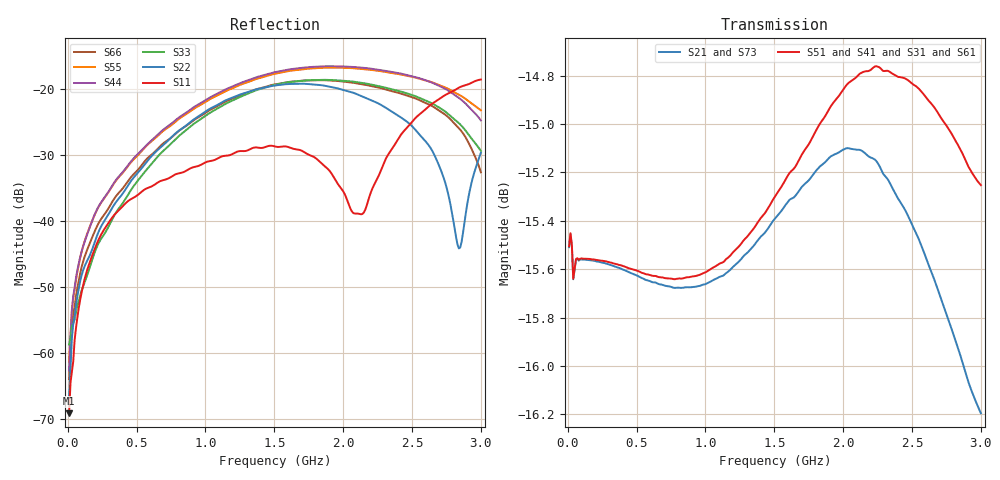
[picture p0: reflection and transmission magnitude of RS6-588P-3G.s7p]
! MTS Systemtechnik GmbH
! S-Parameters
! Model: z.B.: RS6-588P-3G
! Rohde & Schwarz ZVB8 2Ports - Version 3.20 - 1145.1010k08 SN: 100119
! Converted & adapted with MATLAB
!  OUT 2 (Port 3)
!  o
! OUT 1 (Port 2) o  /  MTS  \  o OUT 3 (Port 4)
!  C (Port 1) o--|  RS6-588P-3G  |
! OUT 6 (Port 7) o  \  /  o OUT 4 (Port 5)
!  o
!  OUT 5 (Port 6)
! S7P File: Measurements:
! <S11,S12,S13,S14,S15,S16,S17>,
! <S21,S22,S23,S24,S25,S26,S27>,
! <S31,S32,S33,S34,S35,S36,S37>,
! <S41,S42,S43,S44,S45,S46,S47>,
! <S51,S52,S53,S54,S55,S56,S57>,
! <S61,S62,S63,S64,S65,S66,S67>,
! <S71,S72,S73,S74,S75,S76,S77>:
# HZ  S  DB  R  50.00
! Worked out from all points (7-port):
!   300 points, 10 MHz to 3 GHz, reference 50 ohm
!   strongest paths, dB at 10 MHz, 760 MHz, 1.51 GHz, 2.26 GHz, 3 GHz:
!     S51: -15.5, -15.6, -15.3, -14.8, -15.3
!     S41: -15.5, -15.6, -15.3, -14.8, -15.3
!     S31: -15.5, -15.6, -15.3, -14.9, -15.5
!     S61: -15.5, -15.7, -15.3, -14.8, -15.5
!     S21: -15.5, -15.7, -15.4, -15.2, -16.2
!     S73: -15.5, -15.7, -15.6, -15.2, -15.7
!   lowest |S11| = -69.1 dB at 10 MHz (marker M1), VSWR 1.00, Z = 50 - j0.0133 ohm
!   |S11| at or under -10 dB: start of sweep to end of sweep
